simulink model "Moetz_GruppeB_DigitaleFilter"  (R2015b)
settings: Solver=VariableStepAuto  StartTime=0.0  StopTime=10.0  RelTol=1e-3
libraries: dsparch4 x1, dspsrcs4 x1, powerlib_meascontrol x1

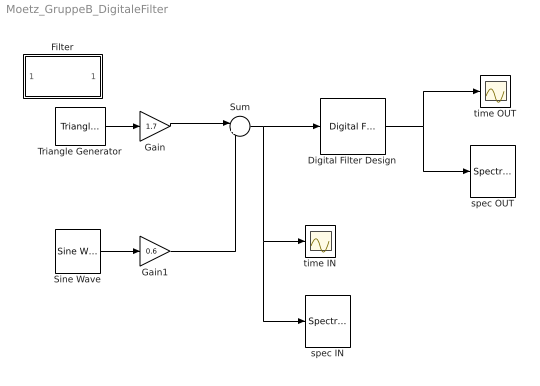
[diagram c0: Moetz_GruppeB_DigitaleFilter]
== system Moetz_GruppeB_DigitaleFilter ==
  Digital Filter Design : dsparch4/Digital Filter Design  mwdsp_browser_bugfix_var=off
  Filter : Subsystem  Tag=FilterWizardSubSystem
  Gain : Gain  Gain=1.7
  Gain1 : Gain  Gain=0.6
  Sine Wave : dspsrcs4/Sine Wave  Amplitude=1  Frequency=110  Phase=0  SampleMode=Discrete  OutComplex=Real  CompMethod=Trigonometric fcn  TableSize=Speed  SampleTime=1/8000  SamplesPerFrame=1  ResetState=Restart at time zero  OutputFrames=off  dataType=double  wordLen=16  udDataType=sfix(16)  fracBitsMode=Best precision  numFracBits=15  OutDataTypeStr=double  LastOutDataTypeStr=double
  Sum : Sum  Inputs=|++
  Triangle Generator : powerlib_meascontrol/Pulse & Signal Generators/Triangle Generator  Freq=14  Phase=90  Ts=1/8000
  spec IN : SpectrumAnalyzer
  spec OUT : SpectrumAnalyzer
  time IN : Scope
  time OUT : Scope
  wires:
  Sine Wave/1 -> Gain1/1
  Triangle Generator/1 -> Gain/1
  Gain/1 -> Sum/1
  Gain1/1 -> Sum/2
  Sum/1 -> spec IN/1, time IN/1, Digital Filter Design/1
  Digital Filter Design/1 -> spec OUT/1, time OUT/1

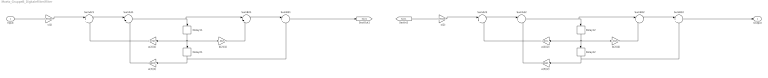
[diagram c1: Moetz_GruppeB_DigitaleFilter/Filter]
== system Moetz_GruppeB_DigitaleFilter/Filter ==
  Input : Inport
  Delay{11..12,21..22} (4 alike) : Delay  DelayLength=1  InitialCondition=0
  SumA{21..22,31..32} (4 alike) : Sum  Inputs=|+-  RndMeth=Nearest
  SumB{21..22,31..32} (4 alike) : Sum  Inputs=|++  RndMeth=Nearest
  a(2)(1) : Gain  Gain=-1.979810101526196  ParamDataTypeStr=double  RndMeth=Nearest
  a(2)(2) : Gain  Gain=-1.9831278714394518  ParamDataTypeStr=double  RndMeth=Nearest
  a(3)(1) : Gain  Gain=0.98825043053133255  ParamDataTypeStr=double  RndMeth=Nearest
  a(3)(2) : Gain  Gain=0.98965857061752782  ParamDataTypeStr=double  RndMeth=Nearest
  b(2)(1) : Gain  Gain=-1.9925342846471645  ParamDataTypeStr=double  RndMeth=Nearest
  b(2)(2) : Gain  Gain=-1.9925342846471645  ParamDataTypeStr=double  RndMeth=Nearest
  s(1) : Gain  Gain=0.99446178813825614  ParamDataTypeStr=double  RndMeth=Nearest
  s(2) : Gain  Gain=0.99446178813825614  ParamDataTypeStr=double  RndMeth=Nearest
  Output : Outport
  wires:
  Input/1 -> s(1)/1
  s(1)/1 -> SumA21/1
  SumA21/1 -> SumA31/1
  SumA31/1 -> SumB21/1, Delay11/1
  SumB21/1 -> SumB31/1
  SumB31/1 -> [Sect1]
  a(2)(1)/1 -> SumA21/2
  Delay11/1 -> a(2)(1)/1, b(2)(1)/1, Delay21/1
  b(2)(1)/1 -> SumB21/2
  a(3)(1)/1 -> SumA31/2
  Delay21/1 -> a(3)(1)/1, SumB31/2
  [Sect1] -> s(2)/1
  s(2)/1 -> SumA22/1
  SumA22/1 -> SumA32/1
  SumA32/1 -> SumB22/1, Delay12/1
  SumB22/1 -> SumB32/1
  SumB32/1 -> Output/1
  a(2)(2)/1 -> SumA22/2
  Delay12/1 -> a(2)(2)/1, b(2)(2)/1, Delay22/1
  b(2)(2)/1 -> SumB22/2
  a(3)(2)/1 -> SumA32/2
  Delay22/1 -> a(3)(2)/1, SumB32/2
